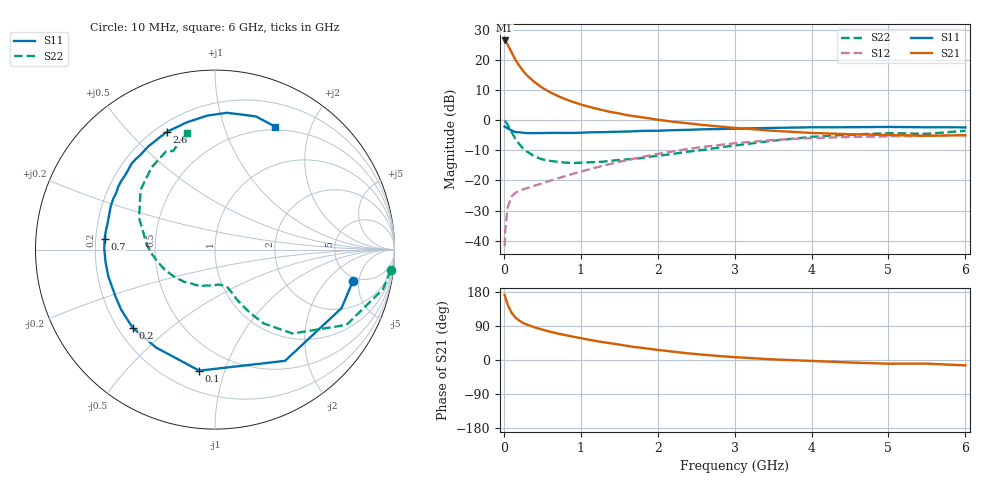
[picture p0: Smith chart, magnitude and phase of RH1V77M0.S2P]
! SIEMENS Small Signal Semiconductors
! BFR106
! Si NPN RF Bipolar Junction Transistor in SOT23
! VCE = 1.75 V  IC = 7 mA
! Common Emitter S-Parameters:  August  1996
# GHz  S  MA  R  50
!  f  S11  S21  S12  S22
! GHz  MAG  ANG  MAG  ANG  MAG  ANG  MAG  ANG
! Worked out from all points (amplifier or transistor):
!   36 points, 10 MHz to 6 GHz, reference 50 ohm
!   highest |S21| = 26.5 dB at 10 MHz (marker M1)
!   |S21| within 3 dB of that: start of sweep to 81.39 MHz
!   unconditionally stable (mu >= 1): 543.2 MHz to 2.334 GHz; 4.287 GHz to end of sweep
!   at 250 MHz: K = 0.61, MSG = 19.7 dB, |S12| = -23.0 dB
!   at 1.4 GHz: K = 1.14, MAG = 6.3 dB, |S12| = -14.4 dB
!   at 6 GHz: K = 1.02, MAG = -1.0 dB, |S12| = -4.8 dB
!   S11 on the Smith chart (normalised r, x): 10 MHz: 4.51, -4.16; 100 MHz: 0.33, -0.82; 200 MHz: 0.26, -0.38; 700 MHz: 0.24, +0.05; 2.6 GHz: 0.24, +0.65; 6 GHz: 0.46, +1.50
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0.01  0.7882 -12.8  21.22 171.8  0.0081 85.5  0.9848 -6.7
0.02  0.7769 -24.8  20.65 165.2  0.016 80.1  0.9622 -13.2
0.05  0.7324 -57.8  18 145.8  0.0358 62.7  0.8441 -29.8
0.1  0.6802 -97.4  13.5 125.2  0.054 48.3  0.636 -47.3
0.15  0.6368 -121.1  10.14 112.0  0.0623 41.3  0.4928 -56.6
0.2  0.6324 -136.5  8.1 104.0  0.0676 39.2  0.4027 -61.0
0.25  0.6209 -147.2  6.615 97.7  0.071 39.0  0.3391 -64.3
0.3  0.6131 -154.5  5.597 93.3  0.0746 39.7  0.303 -66.3
0.4  0.613 -166.0  4.306 86.1  0.0822 42.1  0.2515 -69.0
0.5  0.6138 -173.5  3.475 80.2  0.0897 45.0  0.2238 -71.4
0.6  0.6167 179.9  2.93 74.7  0.0991 47.5  0.2118 -74.1
0.7  0.6182 174.5  2.542 69.9  0.1081 50.0  0.2046 -77.9
0.9  0.6166 165.6  2.014 61.5  0.1294 53.2  0.1951 -85.2
1.1  0.6296 157.2  1.686 53.7  0.1523 55.2  0.2003 -94.6
1.3  0.6352 149.8  1.457 46.8  0.1778 55.7  0.2058 -103.9
1.6  0.6499 140.4  1.22 37.4  0.2177 55.1  0.2244 -118.6
2.2  0.6845 122.9  0.946 22.0  0.3052 49.5  0.2765 -148.1
2.6  0.7093 112.0  0.833 13.8  0.3625 43.5  0.3239 -167.1
3.5  0.7482 93.2  0.67 1.6  0.4704 28.1  0.4582 157.4
4.5  0.7673 78.6  0.587 -6.6  0.5278 11.1  0.5782 127.7
5.5  0.7656 67.4  0.554 -9.6  0.55 1.0  0.5971 113.1
6  0.7627 63.9  0.564 -14.2  0.5748 -6.3  0.6683 103.7
